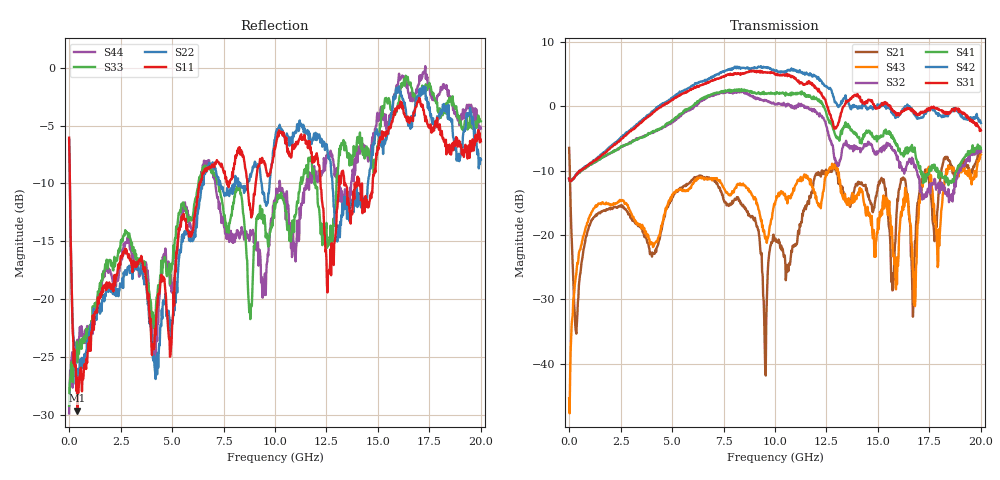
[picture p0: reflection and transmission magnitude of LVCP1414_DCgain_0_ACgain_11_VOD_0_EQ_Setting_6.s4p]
!Agilent Technologies,N5230A,MY46400459,A.07.50.48
!Agilent N5230A: A.07.50.48
!Date: Tuesday, April 17, 2012 18:43:13
!Correction: S11(Full 4 Port(1,2,3,4))
!S12(Full 4 Port(1,2,3,4))
!S13(Full 4 Port(1,2,3,4))
!S14(Full 4 Port(1,2,3,4))
!S21(Full 4 Port(1,2,3,4))
!S22(Full 4 Port(1,2,3,4))
!S23(Full 4 Port(1,2,3,4))
!S24(Full 4 Port(1,2,3,4))
!S31(Full 4 Port(1,2,3,4))
!S32(Full 4 Port(1,2,3,4))
!S33(Full 4 Port(1,2,3,4))
!S34(Full 4 Port(1,2,3,4))
!S41(Full 4 Port(1,2,3,4))
!S42(Full 4 Port(1,2,3,4))
!S43(Full 4 Port(1,2,3,4))
!S44(Full 4 Port(1,2,3,4))
!S4P File: Measurements: <S11,S12,S13,S14>,
!<S21,S22,S23,S24>,
!<S31,S32,S33,S34>,
!<S41,S42,S43,S44>:
# Hz S  dB  R 50
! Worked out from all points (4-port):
!   801 points, 300 kHz to 20 GHz, reference 50 ohm
!   strongest paths, dB at 300 kHz, 5 GHz, 10 GHz, 15 GHz, 20 GHz:
!     S31: -11.2, 1.0, 4.9, -0.3, -3.8
!     S42: -11.4, 1.3, 5.5, 0.2, -2.6
!     S41: -11.3, -2.2, 1.8, -4.7, -6.6
!     S32: -11.3, -2.5, 0.3, -7.3, -7.0
!     S43: -45.3, -13.8, -15.3, -17.4, -7.5
!     S21: -6.5, -14.2, -20.5, -12.3, -7.1
!   lowest |S11| = -29.7 dB at 400.3 MHz (marker M1), VSWR 1.07, Z = 53.1 + j1.38 ohm
!   |S11| at or under -10 dB: 37.58 MHz to 6.325 GHz (6.287 GHz wide, 198 % of centre); 12.21 GHz to 13.11 GHz (897.2 MHz wide, 7.09 % of centre); 14.23 GHz to 14.74 GHz (518.2 MHz wide, 3.58 % of centre)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
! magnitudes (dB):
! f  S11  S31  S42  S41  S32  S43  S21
! 300 kHz  -6.0  -11.2  -11.4  -11.3  -11.3  -45.3  -6.5
! 400.3 MHz  -29.7  -10.4  -10.4  -10.5  -10.5  -24.3  -32.4
! 6.275 GHz  -10.6  3.1  3.6  0.7  0.3  -11.1  -11.0
! 9.525 GHz  -8.3  5.3  6.0  2.0  0.9  -20.6  -40.9
! 12.73 GHz  -17.9  -1.8  2.6  -2.7  -5.4  -9.7  -10.1
! 16.8 GHz  -3.6  -0.9  -1.3  -7.0  -9.1  -31.0  -20.9
! 20 GHz  -6.4  -3.8  -2.6  -6.6  -7.0  -7.5  -7.1
